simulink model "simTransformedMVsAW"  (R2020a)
settings: Solver=ode15s  StartTime=0.0  StopTime=tsim  MaxStep=1  RelTol=1e-3
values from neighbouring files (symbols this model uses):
  d1_step = 60    [runTransformedMVs.m]
  d1nom = T0nom    (= 10)    [runTransformedMVs.m]
  d2_step = d2nom*0.5    (= 0.005)    [runTransformedMVs.m]
  d2nom = qnom    (= 0.01)    [runTransformedMVs.m]
  Kc = 0    [PI_Tank.m]    (also in runCascade.m = tauQ/(tauC+theta); runTransformedMVs.m = 0.01; Main.m = 1/k*tau/(tauC+theta); runTransf.m = 1/kM(i)*tau(i)/(tauCM(i)+theta(i)))
  p = [V;rho;cp;qnom;MV;transf]    [PI_Tank.m]    (also in runCascade.m = [V;rho;cp;A;tau0;MV;transf]; runTransformedMVs.m = [V;rho;cp;A;tau0;MV;transf]; Main.m = [N, Fc0, rhoc, rhoh,U,A,cpc,cph]; Main_OL.m = [N, Fc0, rhoc, rhoh,U,A,cpc,cph])
  tauI = 1    [PI_Tank.m]    (also in runCascade.m = min(tauQ,4*(tauC+theta)); runTransformedMVs.m = 400; Main.m = min(tau,4*(tauC+theta)); runTransf.m = min(tau(i), 4*(tauCM(i)+theta(i))))
  tauT = 400    [runTransformedMVs.m]
  Tnom = 50    [PI_Tank.m]    (also in runCascade.m; runTransformedMVs.m)
  transf = p(7)    [CalcBlock.m]    (also in CalcBlock_num.m; CalcBlock_v.m; PI_Tank.m = j; runCascade.m = j)
  Tstep = Tnom+10    (= 60)    [PI_Tank.m]    (also in runCascade.m = 40; runTransformedMVs.m = -10)
  tstep_d1 = 150    [runTransformedMVs.m]
  tstep_d2 = 20000    [runTransformedMVs.m]
  tstep_T1 = 100    [runTransformedMVs.m]
  umax = inf    [runCascade.m]    (also in runTransformedMVs.m = 5016)
  vbias = Tnom    (= 50)    [runCascade.m]    (also in runTransformedMVs.m = 0)
  vmin = -inf    [runTransformedMVs.m]
undefined symbols (not defined in the file or in its folder): CalcBlock, CalcBlock_v, Tank

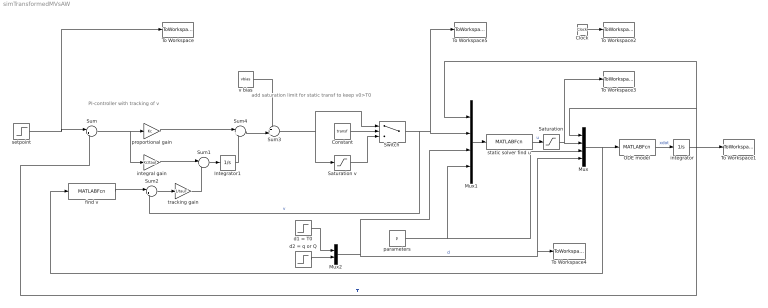
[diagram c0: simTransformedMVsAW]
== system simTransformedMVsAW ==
  note: add saturation limit for static transf to keep v0>T0
  note: PI-controller with tracking of v
  " integrator" : Integrator  InitialCondition=Tnom
  Clock : Clock
  Constant : Constant  Value=transf
  Integrator1 : Integrator
  Mux : Mux
  Mux1 : Mux
  Mux2 : Mux  Inputs=2
  ODE model : MATLABFcn  MATLABFcn=Tank(u(1), u(2),u(3:9),u(10:11))  OutputDimensions=1
  Saturation : Saturate  UpperLimit=umax  LowerLimit=1e-4
  Saturation v : Saturate  UpperLimit=inf  LowerLimit=vmin
  Sum : Sum  Inputs=|+-
  Sum1 : Sum  Inputs=|++
  Sum2 : Sum  Inputs=|+-
  Sum3 : Sum  Inputs=++|
  Sum4 : Sum  Inputs=|++
  Switch : Switch  Criteria=u2 ~= 0
  To Workspace : ToWorkspace  VariableName=Tsp  SampleTime=-1
  To Workspace1 : ToWorkspace  VariableName=T  SampleTime=-1
  To Workspace2 : ToWorkspace  VariableName=time  SampleTime=-1
  To Workspace3 : ToWorkspace  VariableName=u  SampleTime=-1
  To Workspace4 : ToWorkspace  VariableName=d  SampleTime=-1
  To Workspace5 : ToWorkspace  VariableName=v  SampleTime=-1
  d1 = T0 : Step  Time=tstep_d1  Before=d1nom  After=d1_step  SampleTime=0
  d2 = q or Q : Step  Time=tstep_d2  Before=d2nom  After=d2_step  SampleTime=0
  find v : MATLABFcn  MATLABFcn=CalcBlock_v(u(1), u(2),u(3:9),u(10:11))  OutputDimensions=1
  integral gain : Gain  Gain=Kc/tauI  Multiplication=Matrix(K*u)
  parameters : Constant  Value=p
  proportional gain : Gain  Gain=Kc  Multiplication=Matrix(K*u)
  setpoint : Step  Time=tstep_T1  Before=Tnom  After=Tstep  SampleTime=0
  static solver find u : MATLABFcn  MATLABFcn=CalcBlock(u(1),u(2),u(3:4),u(5:11))  OutputDimensions=1
  tracking gain : Gain  Gain=1/tauT  Multiplication=Matrix(K*u)
  v bias : Constant  Value=vbias
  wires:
  " integrator"/1 -> Mux/1, Mux1/1, To Workspace1/1, Sum/2  "T"
  Mux/1 -> find v/1, ODE model/1
  Clock/1 -> To Workspace2/1
  Sum/1 -> integral gain/1, proportional gain/1
  static solver find u/1 -> Saturation/1  "u"
  Sum4/1 -> Sum3/2
  Mux1/1 -> static solver find u/1
  integral gain/1 -> Sum1/1
  proportional gain/1 -> Sum4/1
  Integrator1/1 -> Sum4/2
  Mux2/1 -> To Workspace4/1, Mux/4, Mux1/3  "d"
  parameters/1 -> Mux1/4, Mux/3
  v bias/1 -> Sum3/1
  setpoint/1 -> Sum/1, To Workspace/1
  Sum3/1 -> Saturation v/1, Switch/1
  Saturation/1 -> Mux/2, To Workspace3/1
  Switch/1 -> Sum2/2, Mux1/2, To Workspace5/1  "v"
  Saturation v/1 -> Switch/3
  Constant/1 -> Switch/2
  Sum1/1 -> Integrator1/1
  Sum2/1 -> tracking gain/1
  ODE model/1 -> " integrator"/1  "xdot"
  find v/1 -> Sum2/1
  tracking gain/1 -> Sum1/2
  d1 = T0/1 -> Mux2/1
  d2 = q or Q/1 -> Mux2/2
